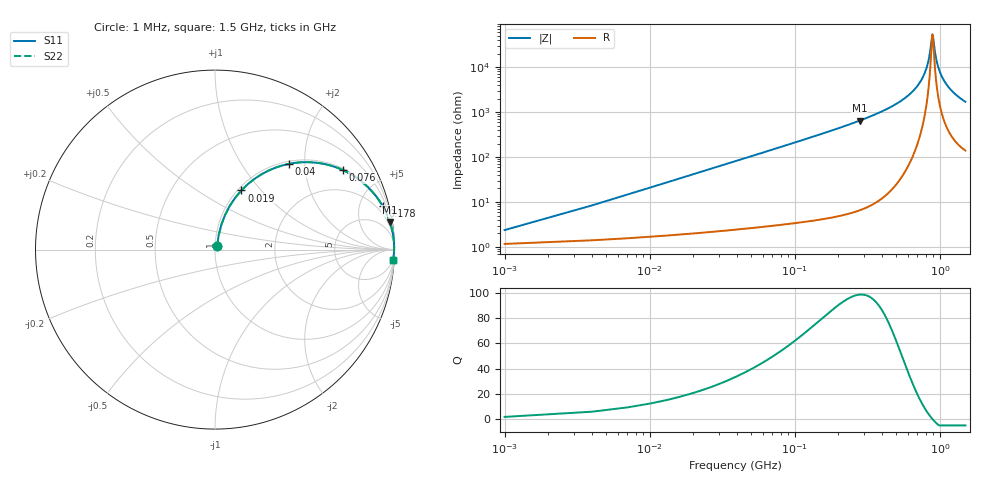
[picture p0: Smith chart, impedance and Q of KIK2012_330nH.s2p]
!version-2
!date-01.2022
!Series
# MHz S RI R 50
!Freq ReS11 ImS11 ReS21 ImS21 ReS12 ImS12 ReS22 ImS22
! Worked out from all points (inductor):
!   501 points, 1 MHz to 1.5 GHz, reference 50 ohm
!   read as one part in series: L = 330 nH near 7 MHz
!   highest Q = 98.5 at 280 MHz (marker M1), where L = 366 nH
!   self-resonance near 889 MHz
!   S11 on the Smith chart (normalised r, x): 1 MHz: 1.02, +0.04; 19 MHz: 1.04, +0.79; 40 MHz: 1.05, +1.66; 76 MHz: 1.06, +3.17; 178 MHz: 1.09, +7.69; 1.5 GHz: 4, -34
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1  0.012 0.0202  0.988 -0.0202  0.988 -0.0202  0.012 0.0202
10  0.0559 0.1925  0.9441 -0.1925  0.9441 -0.1925  0.0559 0.1925
19  0.1468 0.3298  0.8532 -0.3298  0.8532 -0.3298  0.1468 0.3298
40  0.4113 0.4776  0.5887 -0.4776  0.5887 -0.4776  0.4113 0.4776
76  0.7123 0.4432  0.2877 -0.4432  0.2877 -0.4432  0.7123 0.4432
118  0.8576 0.3423  0.1424 -0.3423  0.1424 -0.3423  0.8576 0.3423
178  0.9342 0.2422  0.0658 -0.2422  0.0658 -0.2422  0.9342 0.2422
253  0.9686 0.1694  0.0314 -0.1694  0.0314 -0.1694  0.9686 0.1694
280  0.975 0.1511  0.025 -0.1511  0.025 -0.1511  0.975 0.1511
502  0.9947 0.0651  0.00533 -0.0651  0.00533 -0.0651  0.9947 0.0651
652  0.9976 0.0342  0.00241 -0.0342  0.00241 -0.0342  0.9976 0.0342
751  0.9982 0.0185  0.0018 -0.0185  0.0018 -0.0185  0.9982 0.0185
829  0.9983 0.00773  0.00174 -0.00773  0.00174 -0.00773  0.9983 0.00773
853  0.9982 0.00464  0.00178 -0.00464  0.00178 -0.00464  0.9982 0.00464
889  0.9981 0.000184  0.00187 -0.000184  0.00187 -0.000184  0.9981 0.000184
898  0.9981 -0.000901  0.00191 0.000901  0.00191 0.000901  0.9981 -0.000901
922  0.998 -0.00374  0.002 0.00374  0.002 0.00374  0.998 -0.00374
943  0.9979 -0.00617  0.0021 0.00617  0.0021 0.00617  0.9979 -0.00617
1003  0.9975 -0.0128  0.00246 0.0128  0.00246 0.0128  0.9975 -0.0128
1105  0.9967 -0.0234  0.00327 0.0234  0.00327 0.0234  0.9967 -0.0234
1252  0.9952 -0.0372  0.00483 0.0372  0.00483 0.0372  0.9952 -0.0372
1500  0.9917 -0.0581  0.00825 0.0581  0.00825 0.0581  0.9917 -0.0581
